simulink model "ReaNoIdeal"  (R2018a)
settings: Solver=VariableStepAuto  StartTime=0.0  StopTime=25  RelTol=1e-3
undefined symbols (not defined in the file): b55bc80e74eb, c2e4, ReaNoIdeal, sdiscope

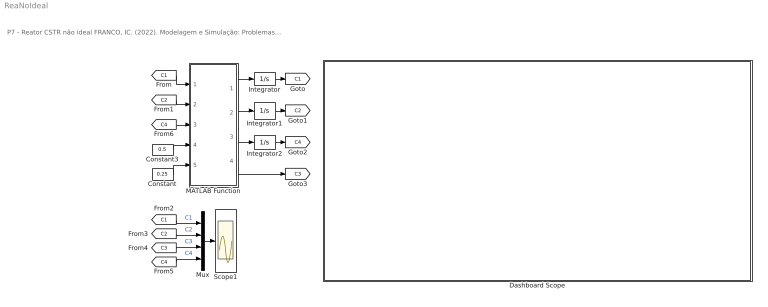
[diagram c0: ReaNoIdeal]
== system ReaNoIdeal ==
  note: P7 - Reator CSTR não ideal FRANCO, IC. (2022). Modelagem e Simulação: Problemas Típicos da Engenharia Química para Simulação e Análise. NOTAS DE AULA INOVADORAS. The Journal of Engineering and Exact Sciences. Material Complementar.
  Constant : Constant  Value=0.25
  Constant3 : Constant  Value=0.5
  Dashboard Scope : Subsystem  DialogController=hmiCreateDDGDialog  IsWebBlock=on  mask(MWDashboardBlock){webBlockId=648504c2-c2e4-4280-8ac4-b55bc80e74eb, webBlockType=sdiscope, ShowInitialText=on, HMISrcModelName=ReaNoIdeal}
      mask prompts: webBlockId "WebBlock Id"; webBlockType "WebBlock Type"; HMISrcModelName "Source Model"
      mask help: SimulinkHMI:dialogs:HMIScopeDialogDesc
  Integrator : Integrator
  Integrator1 : Integrator
  Integrator2 : Integrator
  MATLAB Function : MATLAB Function  TreatAsAtomicUnit=on
  Mux : Mux
  Scope1 : Scope
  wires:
  MATLAB Function/4(C3) -> [C3]
  Constant3/1 -> MATLAB Function/4(f1)
  Constant/1 -> MATLAB Function/5(f2)
  MATLAB Function/2(dC2) -> Integrator1/1
  [C1] -> MATLAB Function/1(C1)
  Integrator/1 -> [C1]
  Integrator1/1 -> [C2]
  [C2] -> MATLAB Function/2(C2)
  MATLAB Function/1(dC1) -> Integrator/1
  MATLAB Function/3(dC4) -> Integrator2/1
  Integrator2/1 -> [C4]
  [C4] -> MATLAB Function/3(C4)
  [C1] -> Mux/1  "C1"
  [C2] -> Mux/2  "C2"
  [C3] -> Mux/3  "C3"
  [C4] -> Mux/4  "C4"
  Mux/1 -> Scope1/1

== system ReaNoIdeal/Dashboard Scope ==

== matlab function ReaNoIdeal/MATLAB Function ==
function [dC1,dC2,dC4,C3] = fcn(C1,C2,C4,f1,f2)
%% Parâmetros
C0    =  1.00;
F     =  1.00;
k     =  0.10;
V     = 10.00;
alpha =  5.00;

%% equações auxiliares
V1 = (1-f2);
V2 = f2*V;
F1 = (1-f1)*F;
F2 = f1*F;
F3 = alpha*F;

%% Modelo matemático
dC1 = (F1/V1)*(C0-C1)+(F3/V1)*(C2-C1)-k*C1;
dC2 = (F3/V2)*(C1-C2)-k*C2;
dC4 = (F/V)*(C0-C4)-k*C4;
C3  = (F1*C1+F2*C0)/F;

end
